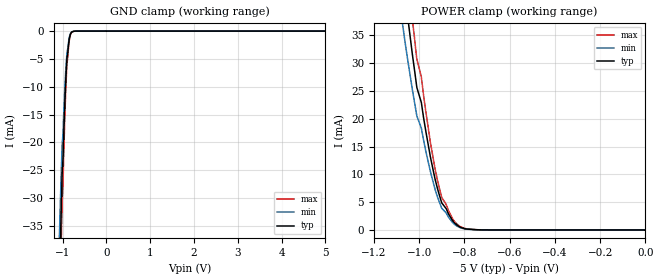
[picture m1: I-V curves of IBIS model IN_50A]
| TEXAS INSTRUMENTS INCORPORATED
| Standard Linear and Logic Group / High Volume Linear
| IBIS Model of TPD4E05U06
| Four Channel ESD Protection Device
| This file contains package information for the following:
|  QFN 10-pin (DQA) package as [Component] TPD4E05U06_DQA
| This device can be powered at the following Vccs:
|  5 volt Vcc
| This file provides unique models under the [Model Selector] for each Vcc.
| For operation at a specific Vcc, select the appropriate model after each
| [Model Selector] keyword.
[IBIS Ver]   3.2
[Comment char]  |_char
[File Name]   tpd4e05u06.ibs
[File Rev]   1.1
[Date]   12/10/2015
[Source]   Data created from TI-SPICE simulations at TI-SLL/HVL.
   The following is an IBIS list for the TPD4E05U06.
   Please contact sllibis@ti.com with questions and
   comments concerning SLL IBIS models.
[Notes]   Revision_History:
|  Rev 1.1   12/10/2015
|  - c comp values revised per PL's request
|  Rev 1.0 October 25, 2012
[Disclaimer]
| This model is designed as an aid for customers of Texas Instruments.
| TI and its licensors and suppliers make no warranties, either expressed
| or implied, with respect to this  model, including the warranties of
| merchantability or fitness for a particular purpose. The model is
| provided solely on an "as is" basis. The entire risk as to its quality
| and performance is with the customer.
[Copyright]
| (C) Copyright 2012 Texas Instruments Incorporated. All rights reserved.
| Component TPD4E05U06_DQA 10-PIN QFN
[Component]   TPD4E05U06_DQA
[Manufacturer]   Texas Instruments, Inc.
[Package]
|   typ   min   max
R_pkg   1.960e-03   1.540e-03   2.470e-03
L_pkg   2.210e-10   1.790e-10   2.640e-10
C_pkg   1.010e-13   7.980e-14   1.280e-13
[Pin]   signal_name   model_name   R_pin   L_pin   C_pin
1   D1P   IN_50A   1.540e-03   1.790e-10   8.040e-14
2   D1N   IN_50A   2.450e-03   2.620e-10   1.280e-13
3   GND   GND   2.450e-03   2.620e-10   1.280e-13
4   D2P   IN_50A   1.540e-03   1.790e-10   8.040e-14
5   D2N   IN_50A   1.780e-03   2.190e-10   9.070e-14
6   NC   NC   1.560e-03   1.800e-10   7.980e-14
7   NC   NC   2.470e-03   2.640e-10   1.270e-13
8   GND   GND   2.470e-03   2.640e-10   1.270e-13
9   NC   NC   1.560e-03   1.800e-10   7.980e-14
10   NC   NC   1.780e-03   2.190e-10   9.070e-14
| Models and submodels in the file (1): IN_50A (Input)
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| Model IN
[Model]   IN_50A
Model_type  Input
Vinl=0
Vinh=5
| variable   typ   min   max
C_comp   0.372pF   0.272pF   0.672pF
[Temperature Range]   40   100   -40
| Ambient temperature   25   85   -40
[Voltage range]   5   5   5
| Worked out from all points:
|   GND clamp passes 1 mA (typ) near -0.84 V on its own axis
|   POWER clamp passes 1 mA (typ) near -0.84 V on its own axis
[GND Clamp]
| IN_50A
| Voltage   I(typ)   I(min)   I(max)
-5V       -1.23A     -985mA     -1.48A
-1.07V    -45.16mA   -36.1mA    -54.2mA
-1.05V    -38.18mA   -30.5mA    -45.8mA
-1.03V    -31.67mA   -25.3mA    -38mA
-1.02V    -28.68mA   -22.9mA    -34.4mA
-1.01V    -25.62mA   -20.5mA    -30.7mA
-990mV    -22.9mA    -18.3mA    -27.5mA
-950mV    -13.12mA   -10.5mA    -15.7mA
-900mV    -4.871mA   -3.9mA     -5.84mA
-850mV    -1.552mA   -1.24mA    -1.86mA
-790mV    -170.1uA   -136uA     -204uA
5V        247pA      198pA      296pA
[POWER Clamp]
| IN_50A
|Voltage   I(typ)   I(min)   I(max)
-5V       1.23A      985mA      1.48A
-1.07V    45.16mA    36.1mA     54.2mA
-1.05V    38.18mA    30.5mA     45.8mA
-1.03V    31.67mA    25.3mA     38mA
-1.02V    28.68mA    22.9mA     34.4mA
-1.01V    25.62mA    20.5mA     30.7mA
-990mV    22.9mA     18.3mA     27.5mA
-950mV    13.12mA    10.5mA     15.7mA
-920mV    7.63mA     6.1mA      9.16mA
-900mV    4.871mA    3.9mA      5.84mA
-830mV    797.3uA    638uA      957uA
0V        0A         0A         0A
